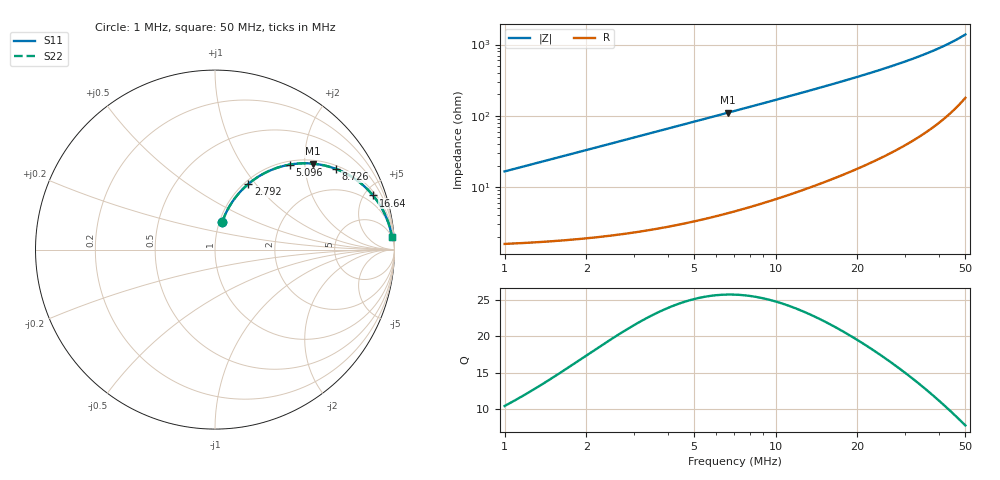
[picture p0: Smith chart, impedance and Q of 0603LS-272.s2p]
# MHz S MA R 50
!Freq  MagS11  AngS11  MagS21  AngS21  MagS12  AngS12  MagS22  AngS22
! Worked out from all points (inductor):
!   801 points, 1 MHz to 50 MHz, reference 50 ohm
!   read as one part in series: L = 2.62 uH near 1.02 MHz
!   highest Q = 25.8 at 6.636 MHz (marker M1), where L = 2.64 uH
!   S11 on the Smith chart (normalised r, x): 1 MHz: 1.03, +0.33; 2.792 MHz: 1.04, +0.92; 5.096 MHz: 1.07, +1.68; 8.726 MHz: 1.11, +2.91; 16.64 MHz: 1.27, +5.73; 50 MHz: 5, +27
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1  0.1607 75.3  0.9717 -9.2  0.9717 -9.2  0.1607 75.3
1.360799  0.2158 73.3  0.9604 -12.4  0.9604 -12.4  0.2158 73.3
1.763399  0.2748 70.5  0.9445 -15.9  0.9445 -15.9  0.2748 70.5
2.240849  0.3408 67.0  0.922 -19.9  0.922 -19.9  0.3408 67.0
2.792413  0.411 63.0  0.8922 -24.2  0.8922 -24.2  0.411 63.0
3.281422  0.4675 59.6  0.8634 -27.8  0.8634 -27.8  0.4675 59.6
3.818539  0.5234 56.0  0.8302 -31.5  0.8302 -31.5  0.5234 56.0
5.095611  0.6321 48.6  0.7502 -39.2  0.7502 -39.2  0.6321 48.6
6.635547  0.7262 41.3  0.6599 -46.5  0.6599 -46.5  0.7262 41.3
7.64653  0.7714 37.3  0.607 -50.4  0.607 -50.4  0.7714 37.3
8.725788  0.8093 33.8  0.5564 -54.0  0.5564 -54.0  0.8093 33.8
9.208004  0.8234 32.4  0.5357 -55.4  0.5357 -55.4  0.8234 32.4
10.76773  0.8601 28.4  0.4761 -59.2  0.4761 -59.2  0.8601 28.4
12.46912  0.8888 24.9  0.4221 -62.6  0.4221 -62.6  0.8888 24.9
14.43933  0.9123 21.7  0.3708 -65.7  0.3708 -65.7  0.9123 21.7
16.63929  0.9307 18.9  0.3245 -68.4  0.3245 -68.4  0.9307 18.9
17.38794  0.9357 18.1  0.3109 -69.2  0.3109 -69.2  0.9357 18.1
21.04132  0.9535 14.8  0.2555 -72.2  0.2555 -72.2  0.9535 14.8
25.58712  0.9667 11.8  0.2051 -74.8  0.2051 -74.8  0.9667 11.8
33.81217  0.9791 8.2  0.1432 -77.5  0.1432 -77.5  0.9791 8.2
41.92918  0.9851 5.8  0.1019 -78.7  0.1019 -78.7  0.9851 5.8
50  0.9883 4.1  0.0713 -78.5  0.0713 -78.5  0.9883 4.1
